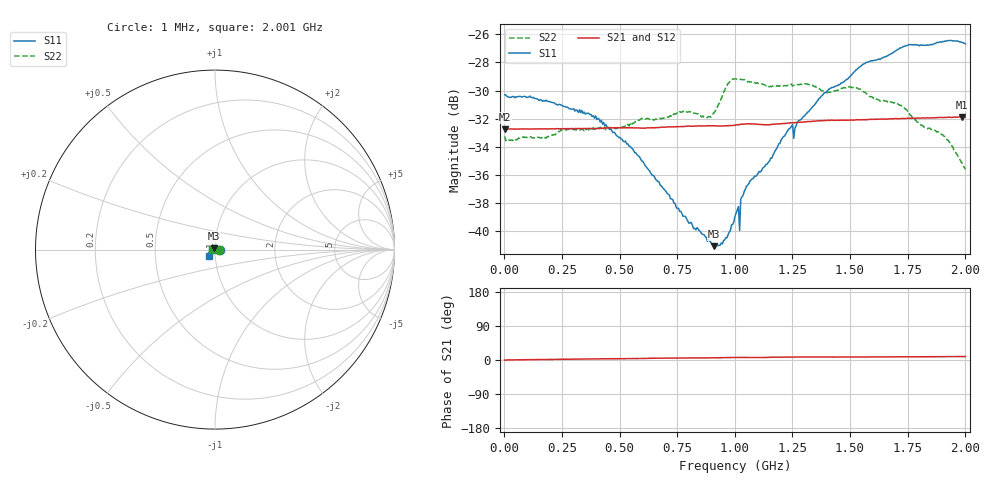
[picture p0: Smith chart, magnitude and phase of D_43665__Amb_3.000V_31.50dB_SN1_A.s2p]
! device id: 43665_
! dir: \\malibu\benchdata\1_engineers\tn_data\43665_75ohm\new\sparar\43665_\amb\3p000v\31p50db
! Serial: 1
! Insertion: A
! Temp: Amb
! VDD: 3.000V
! Attenuation Step: 31.50dB
! IDD: 1.454096e+00mA
! FILE NAME
! DATE 03-27-2009 08:42:22
! CORRECTED  DATA
#  Hz  S  RI  R  75
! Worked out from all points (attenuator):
!   401 points, 1 MHz to 2.001 GHz, reference 75 ohm
!   highest |S21| = -31.88 dB at 1.986 GHz (marker M1); lowest = -32.8 dB at 1 MHz (marker M2)
!   lowest |S11| = -41.1 dB at 911 MHz (marker M3), VSWR 1.02, Z = 74.4 + j1.17 ohm
!   |S11| at or under -10 dB: start of sweep to end of sweep
!   |S22| runs from -35.6 to -29.2 dB; largest |S21 - S12| = 0.00015
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1000000  0.0305 -0.000133  0.023 -7.78e-05  0.023 5.9e-05  0.0217 6.48e-08
3.36e8  0.0257 0.00798  0.0231 0.00097  0.0232 0.00099  0.0125 0.0194
5.36e8  0.0172 0.011  0.0233 0.00147  0.0233 0.00149  0.00165 0.0239
6.71e8  0.0101 0.0111  0.0233 0.00194  0.0233 0.00196  -0.00701 0.024
8.11e8  0.00254 0.0104  0.0235 0.0022  0.0235 0.00228  -0.0157 0.0211
8.76e8  -0.00171 0.00932  0.0236 0.00234  0.0236 0.0024  -0.0189 0.0169
9.11e8  -0.00404 0.00783  0.0235 0.00241  0.0235 0.00245  -0.0219 0.0148
9.56e8  -0.00643 0.0067  0.0235 0.00254  0.0236 0.00258  -0.0283 0.0143
1.001e9  -0.00923 0.00645  0.0236 0.00276  0.0237 0.00279  -0.0308 0.0163
1.061e9  -0.0136 0.00557  0.0239 0.00277  0.0239 0.0028  -0.0309 0.0143
1.151e9  -0.0176 0.00229  0.0237 0.00293  0.0237 0.00302  -0.0308 0.0108
1.241e9  -0.0232 -0.00157  0.0241 0.00322  0.024 0.00329  -0.0324 0.00627
1.266e9  -0.0234 -0.00328  0.0241 0.0033  0.0241 0.00333  -0.0327 0.00474
1.336e9  -0.0269 -0.00591  0.0243 0.00339  0.0244 0.00344  -0.0329 0.00234
1.401e9  -0.0298 -0.00993  0.0245 0.00341  0.0245 0.00344  -0.031 -0.000976
1.551e9  -0.0347 -0.0176  0.0246 0.00344  0.0247 0.0035  -0.0313 -0.00564
1.671e9  -0.0357 -0.023  0.0248 0.00365  0.0249 0.00366  -0.0282 -0.00621
1.746e9  -0.0362 -0.0279  0.0249 0.00367  0.025 0.0037  -0.0257 -0.00837
1.811e9  -0.0345 -0.0302  0.0249 0.00375  0.025 0.00375  -0.0227 -0.00704
1.901e9  -0.0345 -0.0324  0.025 0.00387  0.0251 0.00394  -0.0211 -0.00654
1.986e9  -0.0318 -0.0345  0.0251 0.00401  0.0252 0.00397  -0.0166 -0.00532
2.001e9  -0.0313 -0.0342  0.0251 0.00404  0.0252 0.00399  -0.016 -0.00443
